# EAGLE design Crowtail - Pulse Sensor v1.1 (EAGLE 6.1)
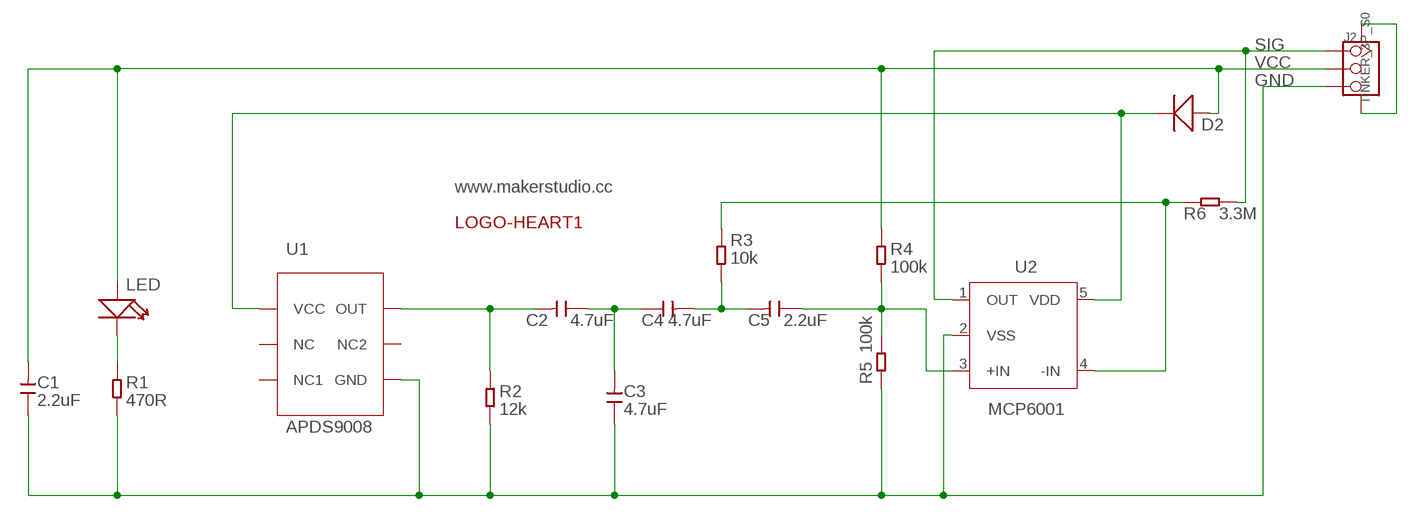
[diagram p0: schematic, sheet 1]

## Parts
C1  2.2uF  C-0603  [0603]
C2  4.7uF  C-0603  [0603]
C3  4.7uF  C-0603  [0603]
C4  4.7uF  C-0603  [0603]
C5  2.2uF  C-0603  [0603]
D2  D'0603'  [SOD523]
J2  TINKER_3P_S0  [TINKER_3P_S0]
L1  LOGO-HEART1  [HEART-1]
LED  LED-AM2520ZGC09  [LED-AM2520ZGC09]
R1  470R  R-0603  [0603]
R2  12k  R-0603  [0603]
R3  10k  R-0603  [0603]
R4  100k  R-0603  [0603]
R5  100k  R-0603  [0603]
R6  3.3M  R-0603  [0603]
U1  APDS9008  APDS-9008  [APDS-9008]
U2  MCP6001  [SOT23-5]

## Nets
GND: C1.1 C3.1 J2.3 J2.SS1 J2.SS2 R1.1 R2.1 R5.1 U1.4(GND) U2.2(VSS)
N$4: LED.2(-) R1.2
N$5: D2.- U1.1(VCC) U2.5(VDD)
N$6: C2.2 R2.2 U1.6(OUT)
N$7: C2.1 C3.2 C4.1
N$8: C4.2 C5.2 R3.1
N$9: C5.1 R4.1 R5.2 U2.3(+IN)
N$10: R3.2 R6.1 U2.4(-IN)
SIG: J2.1 R6.2 U2.1(OUT)
VCC: C1.2 D2.+ J2.2 LED.1(+) R4.2
Unconnected: U1.2(NC) U1.3(NC1) U1.5(NC2)

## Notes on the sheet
- www.makerstudio.cc

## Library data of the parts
C1-C5 = Discrete:C*: Ceramic Capacitors
D2 = Discrete:D*
J2 = Connector:TINKER_3P_S0
L1 = Logo:LOGO-HEART1
LED = Discrete:LED-AM2520ZGC09
R1-R6 = Discrete:R*
U1 = IC:APDS-9008
U2 = IC:MCP6001

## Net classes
0 default: width 0.203 mm, drill 0.305 mm, clearance 0.203 mm

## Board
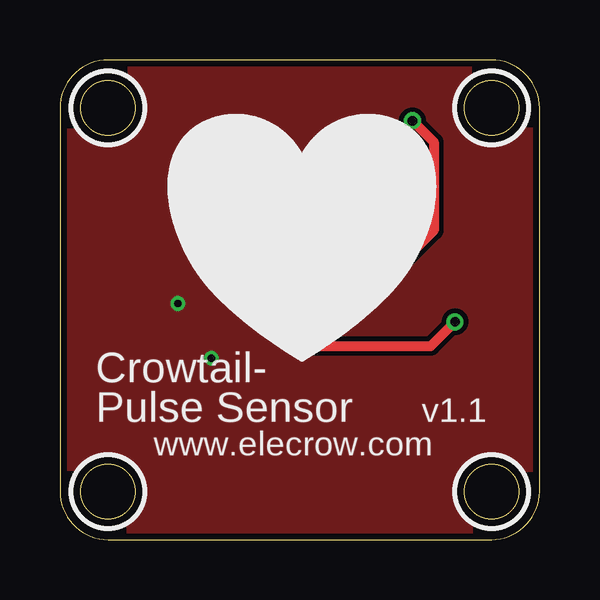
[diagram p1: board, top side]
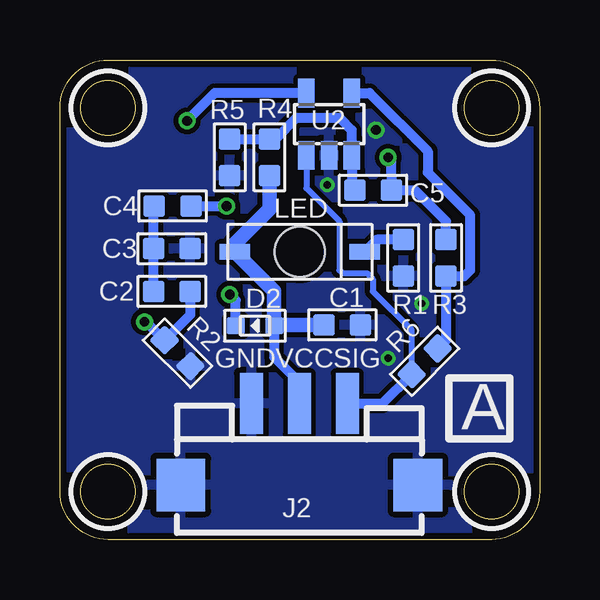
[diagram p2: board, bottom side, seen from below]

Size 20 x 20 mm. Coordinates in mm from the lower left corner, seen from the top.
Outline: 20,2 20,18 arc90 18,20 2,20 arc90 0,18 0,2 arc90 2,0 18,0 arc90 20,2
Outline: circle at 18,2 radius 1.14
Outline: circle at 2,2 radius 1.14
Outline: circle at 18,18 radius 1.14
Outline: circle at 2,18 radius 1.14
Copper layers (1*16): Top 0.035mm / dielectric 1.5mm / Bottom 0.035mm
Design rules: minimum track width 6mil, minimum drill 12mil, track to track 6mil, track to pad 6mil, pad to pad 6mil, via to via 6mil, smd to smd 0mil, copper to edge 10mil, drill to drill 10mil, minimum pad ring 10mil, minimum via ring 6mil, stop-mask expansion 2mil, vias tented up to drill 100mil, thermal gap 10mil
tRestrict: area 16.5,0.5 to 19.5,3.5; area 0.5,0.5 to 3.5,3.5; area 16.5,16.5 to 19.5,19.5; area 0.5,16.5 to 3.5,19.5
bRestrict: area 16.5,0.5 to 19.5,3.5; area 0.5,0.5 to 3.5,3.5; area 16.5,16.5 to 19.5,19.5; area 0.5,16.5 to 3.5,19.5

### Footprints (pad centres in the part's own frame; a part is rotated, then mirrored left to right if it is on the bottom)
0603 = smd 0.889 x 0.889: 1 -0.762,0; 2 0.762,0
SOD523 = smd 0.762 x 0.7: + -0.8,0; - 0.8,0
TINKER_3P_S0 = smd 0.965 x 2.54: 1 -1.984,-3.175; 2 0.016,-3.175; 3 2.016,-3.175 | smd 2.032 x 2.184: SS1 -4.93,0.225; SS2 4.962,0.225
LED-AM2520ZGC09 = smd 1.27 x 0.635: 1 -2.7,0; 2 2.7,0 | hole 2.1: 0,0
APDS-9008 = smd 0.45 x 0.5: 1 0.678,0.723; 3 -0.672,0.723; 4 -0.672,-0.723; 6 0.678,-0.723 | smd 0.4 x 0.5: 2 -0.002,0.723; 5 -0.002,-0.723
SOT23-5 = smd 0.69 x 1.2: 1 -0.95,-1.3; 2 0,-1.3; 3 0.95,-1.3; 4 0.95,1.3; 5 -0.95,1.3

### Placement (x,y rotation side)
C1  8.22,8.95 180 bottom
C2  15.33,10.35 0 bottom
C3  15.33,12.13 180 bottom
C4  15.3,13.91 0 bottom
C5  6.94,14.57 0 bottom
D2  11.87,8.92 180 bottom
J2  10,2.5 180 bottom
L1  10,12.5 0 top
LED  10,12 0 bottom
R1  5.68,11.75 90 bottom
R2  15.09,7.77 135 bottom
R3  3.9,11.75 270 bottom
R4  11.27,15.94 270 bottom
R5  12.92,15.94 90 bottom
R6  4.79,7.43 225 bottom
U1  10,9.87 270 top
U2  8.78,17.32 0 bottom

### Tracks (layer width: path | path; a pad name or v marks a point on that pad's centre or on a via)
GND  (via drill 0.3, 0.41)
  other vias: 6.82,17.08 8.86,14.79 6.32,7.56 4.92,9.84
  pour Top: 0.5,-1.5 19.5,-1.5 arc90 21.5,0.5 21.5,19.5 arc90 19.5,21.5 0.5,21.5 arc90 -1.5,19.5 -1.5,0.5 arc90
  pour Bottom: 1,-1 19,-1 arc90 21,1 21,19 arc90 19,21 1,21 arc90 -1,19 -1,1 arc90
N$4
  Bottom 0.406: R1.2 6.79,12.51 LED.2
N$5  (via drill 0.41 pad 0.41)
  Top 0.406: U1.1 11.89,9.2 v12.92,10.22 15.59,12.89 15.59,16.57 v14.7,17.46
  Bottom 0.406: U2.5 13.54,18.62 v14.7,17.46 | D2.- 12.67,9.97 v12.92,10.22 12.98,10.29
N$6  (via drill 0.41 pad 0.41)
  Top 0.406: U1.6 9.28,8.79 10.13,8.06 15.46,8.06 v16.48,9.08
  Bottom 0.406: C2.2 14.57,9.37 R2.2 16.4,9.08 v16.48,9.08
N$7
  Bottom 0.406: C2.1 C3.2 16.09,13.88 C4.1
N$8  (via drill 0.41 pad 0.41)
  Top 0.406: v13.05,13.91 8.22,13.91 v6.32,15.94
  Bottom 0.254: 12.92,13.91 v13.05,13.91
  Bottom 0.406: C4.2 12.92,13.91 | v6.32,15.94 6.19,15.83 C5.2 5.2,14.57 3.9,13.27 R3.1
N$9
  Bottom 0.406: C5.1 7.83,14.83 U2.3 7.84,17.08 8.35,17.59 10.13,17.59 11.02,16.7 R4.1 R5.2
N$10
  Bottom 0.406: U2.4 7.09,18.62 4.67,16.19 4.67,15.3 2.89,13.53 2.89,11.24 3.14,10.98 R3.2 3.9,8.32 R6.1
SIG
  Bottom 0.254: U2.1 9.73,14.65 8.35,13.27 8.35,11.24 8.22,11.11 7.21,11.11 6.95,10.86 6.95,10.35 5.33,8.73 R6.2
  Bottom 0.406: J2.1 6.55,5.67 R6.2
VCC
  Bottom 0.406: D2.+ 11.07,7.61 10,6.54 10,5.69 J2.2
  Bottom 0.61: R4.2 11.27,13.78 12.7,12.35 LED.1 11.07,10.37 D2.+ 11.03,8.95 C1.2

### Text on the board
tPlace: Crowtail- | Pulse Sensor | v1.1 | www.elecrow.com
bPlace: SIG | VCC | GND | A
